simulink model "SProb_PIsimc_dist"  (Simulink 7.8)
settings: Solver=ode3  StartTime=0.0  StopTime=50  FixedStep=0.01  RelTol=1e-7
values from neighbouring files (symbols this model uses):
  delay = delayv(i)    [example.m]    (also in IAE_Simulink.m; Robustness_SP.m; Robustness_SP_P.m; Robustness_SP_PI.m)
libraries: simulink x2

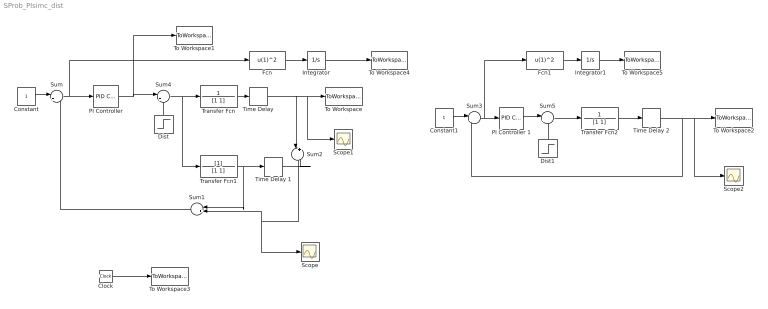
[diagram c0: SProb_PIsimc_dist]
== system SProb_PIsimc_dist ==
  Clock : Clock
  Constant : Constant
  Constant1 : Constant
  Dist : Step  Time=0  SampleTime=0
  Dist1 : Step  Time=0  SampleTime=0
  Fcn : Fcn  Expr=u(1)^2
  Fcn1 : Fcn  Expr=u(1)^2
  Integrator : Integrator
  Integrator1 : Integrator
  PI Controller : simulink/Continuous/PID Controller  Controller=PI  TimeDomain=Continuous-time  SampleTime=1  IntegratorMethod=Forward Euler  FilterMethod=Forward Euler  Form=Ideal  P=4  I=1  D=0  N=100  InitialConditionSource=internal  InitialConditionForIntegrator=0  InitialConditionForFilter=0  ExternalReset=none  LimitOutput=off  UpperSaturationLimit=inf  LowerSaturationLimit=-inf  LinearizeAsGain=off  AntiWindupMode=none  Kb=1  TrackingMode=off  Kt=1  PParamMin=[]  PParamMax=[]  IParamMin=[]  IParamMax=[]  DParamMin=[]  DParamMax=[]  NParamMin=[]  NParamMax=[]  KbParamMin=[]  KbParamMax=[]  KtParamMin=[]  KtParamMax=[]  POutMin=[]  POutMax=[]  IOutMin=[]  IOutMax=[]  DOutMin=[]  DOutMax=[]  NOutMin=[]  NOutMax=[]  KbOutMin=[]  KbOutMax=[]  KtOutMin=[]  KtOutMax=[]  IntegratorOutMin=[]  IntegratorOutMax=[]  FilterOutMin=[]  FilterOutMax=[]  SumOutMin=[]  SumOutMax=[]  SumI1OutMin=[]  SumI1OutMax=[]  SumI2OutMin=[]  SumI2OutMax=[]  SumI3OutMin=[]  SumI3OutMax=[]  SumDOutMin=[]  SumDOutMax=[]  SaturationOutMin=[]  SaturationOutMax=[]  IntegratorContinuousStateAttributes=''  IntegratorStateMustResolveToSignalObject=off  IntegratorRTWStateStorageClass=Auto  FilterContinuousStateAttributes=''  FilterStateMustResolveToSignalObject=off  FilterRTWStateStorageClass=Auto
  PI Controller 1 : simulink/Continuous/PID Controller  Controller=PI  TimeDomain=Continuous-time  SampleTime=1  IntegratorMethod=Forward Euler  FilterMethod=Forward Euler  Form=Ideal  P=0.5  I=1  D=0  N=100  InitialConditionSource=internal  InitialConditionForIntegrator=0  InitialConditionForFilter=0  ExternalReset=none  LimitOutput=off  UpperSaturationLimit=inf  LowerSaturationLimit=-inf  LinearizeAsGain=off  AntiWindupMode=none  Kb=1  TrackingMode=off  Kt=1  PParamMin=[]  PParamMax=[]  IParamMin=[]  IParamMax=[]  DParamMin=[]  DParamMax=[]  NParamMin=[]  NParamMax=[]  KbParamMin=[]  KbParamMax=[]  KtParamMin=[]  KtParamMax=[]  POutMin=[]  POutMax=[]  IOutMin=[]  IOutMax=[]  DOutMin=[]  DOutMax=[]  NOutMin=[]  NOutMax=[]  KbOutMin=[]  KbOutMax=[]  KtOutMin=[]  KtOutMax=[]  IntegratorOutMin=[]  IntegratorOutMax=[]  FilterOutMin=[]  FilterOutMax=[]  SumOutMin=[]  SumOutMax=[]  SumI1OutMin=[]  SumI1OutMax=[]  SumI2OutMin=[]  SumI2OutMax=[]  SumI3OutMin=[]  SumI3OutMax=[]  SumDOutMin=[]  SumDOutMax=[]  SaturationOutMin=[]  SaturationOutMax=[]  IntegratorContinuousStateAttributes=''  IntegratorStateMustResolveToSignalObject=off  IntegratorRTWStateStorageClass=Auto  FilterContinuousStateAttributes=''  FilterStateMustResolveToSignalObject=off  FilterRTWStateStorageClass=Auto
  Scope : Scope
  Scope1 : Scope
  Scope2 : Scope
  Sum : Sum  Inputs=|+-
  Sum1 : Sum  Inputs=|++
  Sum2 : Sum  Inputs=|+-
  Sum3 : Sum  Inputs=|+-
  Sum4 : Sum  Inputs=|++
  Sum5 : Sum  Inputs=|++
  Time Delay : TransportDelay  DelayTime=delay
  Time Delay 1 : TransportDelay
  Time Delay 2 : TransportDelay  DelayTime=delay
  To Workspace : ToWorkspace  VariableName=Ysp  SampleTime=-1  SaveFormat=Array
  To Workspace1 : ToWorkspace  VariableName=usp  SampleTime=-1  SaveFormat=Structure
  To Workspace2 : ToWorkspace  VariableName=Ypi  SampleTime=-1  SaveFormat=Array
  To Workspace3 : ToWorkspace  VariableName=time  SampleTime=-1  SaveFormat=Array
  To Workspace4 : ToWorkspace  VariableName=ISE_SP2  SampleTime=-1  SaveFormat=Array
  To Workspace5 : ToWorkspace  VariableName=ISE_IP  SampleTime=-1  SaveFormat=Array
  Transfer Fcn : TransferFcn  Numerator=1  Denominator=[1 1]
  Transfer Fcn1 : TransferFcn  Denominator=[1 1]
  Transfer Fcn2 : TransferFcn  Numerator=1  Denominator=[1 1]
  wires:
  Constant/1 -> Sum/1
  Sum/1 -> PI Controller/1, Fcn/1
  PI Controller/1 -> To Workspace1/1, Sum4/1
  Transfer Fcn/1 -> Time Delay/1
  Transfer Fcn1/1 -> Time Delay 1/1, Sum1/1
  Time Delay/1 -> Sum2/1, To Workspace/1, Scope1/1
  Time Delay 1/1 -> Sum2/2
  Sum2/1 -> Sum1/2, Scope/1
  Sum1/1 -> Sum/2
  Transfer Fcn2/1 -> Time Delay 2/1
  Sum3/1 -> PI Controller 1/1, Fcn1/1
  Constant1/1 -> Sum3/1
  Time Delay 2/1 -> Sum3/2, To Workspace2/1, Scope2/1
  Clock/1 -> To Workspace3/1
  Sum4/1 -> Transfer Fcn/1, Transfer Fcn1/1
  Dist/1 -> Sum4/2
  PI Controller 1/1 -> Sum5/1
  Dist1/1 -> Sum5/2
  Sum5/1 -> Transfer Fcn2/1
  Fcn/1 -> Integrator/1
  Integrator/1 -> To Workspace4/1
  Fcn1/1 -> Integrator1/1
  Integrator1/1 -> To Workspace5/1
